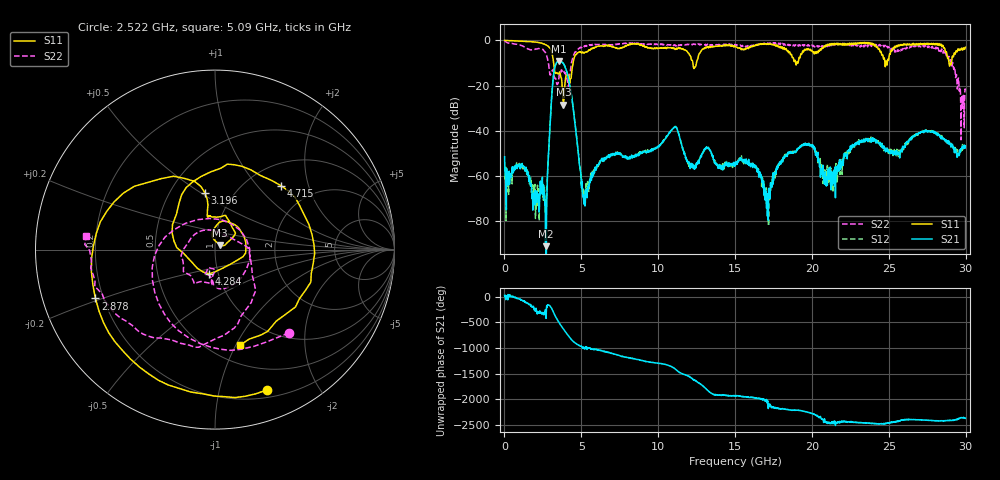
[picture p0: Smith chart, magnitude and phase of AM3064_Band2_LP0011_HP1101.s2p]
# Hz S DB R 50.0
!freq dBS11 angS11 dBS21 angS21 dBS12 angS12 dBS22 angS22
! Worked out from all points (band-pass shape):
!   1600 points, 10 MHz to 29.98 GHz, reference 50 ohm
!   highest |S21| = -9.09 dB at 3.534 GHz (marker M1); lowest = -91.1 dB at 2.672 GHz (marker M2)
!   |S21| within 3 dB of the highest: 3.268 GHz to 3.959 GHz (691.1 MHz wide, 19.1 % of centre)
!   lowest |S11| = -28.4 dB at 3.834 GHz (marker M3), VSWR 1.08, Z = 52.7 + j2.77 ohm
!   |S11| at or under -10 dB: 3.199 GHz to 4.465 GHz (1.267 GHz wide, 33.1 % of centre); 12.26 GHz to 12.49 GHz (233.3 MHz wide, 1.89 % of centre); 28.91 GHz to 29.08 GHz (164.8 MHz wide, 0.569 % of centre)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
!   |S22| runs from -44.0 to -0.2 dB; largest |S21 - S12| = 0.012
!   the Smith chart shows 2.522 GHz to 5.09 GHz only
!   S11 on the Smith chart (normalised r, x): 2.522 GHz: 0.27, -1.40; 2.878 GHz: 0.17, -0.19; 3.196 GHz: 0.74, +0.52; 4.284 GHz: 0.90, -0.25; 4.715 GHz: 1.41, +1.36; 5.09 GHz: 0.68, -1.04
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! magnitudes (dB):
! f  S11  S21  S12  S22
! 10 MHz  -0.1  -51.5  -61.2  -0.2
! 2.522 GHz  -1.6  -66.4  -70.7  -4.2
! 2.672 GHz  -2.0  -91.1  -70.1  -5.5
! 2.878 GHz  -2.9  -48.8  -48.4  -10.9
! 3.196 GHz  -9.9  -15.1  -15.1  -13.9
! 3.534 GHz  -14.7  -9.1  -9.3  -17.0
! 3.834 GHz  -28.4  -10.3  -10.2  -13.4
! 4.284 GHz  -17.2  -21.2  -21.0  -13.7
! 4.715 GHz  -5.8  -44.2  -44.0  -4.3
! 5.015 GHz  -5.6  -65.3  -61.4  -3.2
! 5.09 GHz  -5.2  -69.3  -66.1  -2.8
! 10 GHz  -3.5  -46.8  -47.1  -1.8
! 11.11 GHz  -4.1  -38.2  -38.1  -2.2
! 12.21 GHz  -8.9  -56.3  -54.8  -2.0
! 15 GHz  -2.5  -55.6  -55.1  -1.9
! 17.12 GHz  -1.7  -74.2  -75.8  -1.2
! 19.99 GHz  -4.4  -46.7  -46.9  -2.1
! 21.38 GHz  -1.4  -59.9  -63.8  -2.1
! 22.95 GHz  -1.2  -45.1  -44.7  -2.4
! 25 GHz  -8.2  -49.1  -48.3  -2.8
! 28.56 GHz  -3.1  -43.5  -43.7  -4.6
! 29.98 GHz  -3.1  -46.8  -47.3  -21.8
